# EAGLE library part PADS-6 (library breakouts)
PIN HEADER
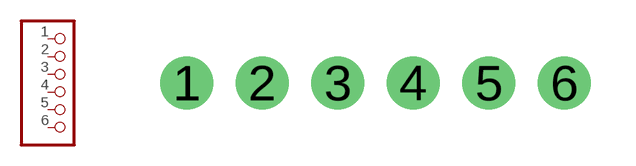
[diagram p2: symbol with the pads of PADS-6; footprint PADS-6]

Designator prefix JP

## PADS-6  [PADS-6]
1  1  pas
2  2  pas
3  3  pas
4  4  pas
5  5  pas
6  6  pas

## Footprint PADS-6 (pad centres in mm)
drill 1.016 pad 1.778: 1 -6.35,0; 2 -3.81,0; 3 -1.27,0; 4 1.27,0; 5 3.81,0; 6 6.35,0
